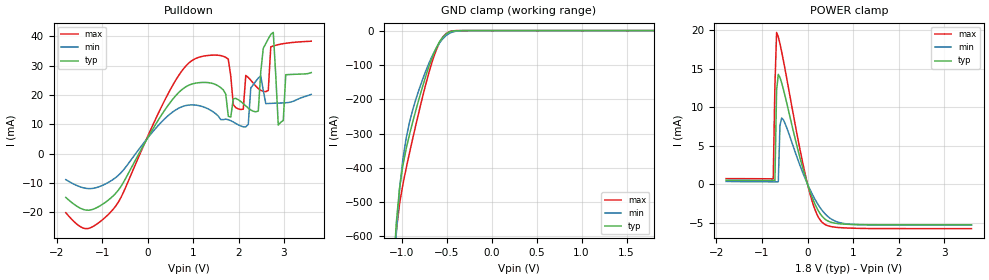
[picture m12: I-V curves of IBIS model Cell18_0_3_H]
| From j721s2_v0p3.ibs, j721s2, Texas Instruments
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|   Model Cell18_0_3_H
[Model]  Cell18_0_3_H
Model_type I/O_open_drain
Polarity   Non-Inverting
Enable   Active-High
Vinl =  0.540V
Vinh =  1.260V
Vmeas =  0.900V
Cref =  50.000pF
Rref =  1.000M
Vref =  0.0V
C_comp   8.808pF   8.664pF   8.912pF
[Model Spec]
Vinh   1.260V   1.134V   1.386V
Vinl   0.540V   0.486V   0.594V
Vmeas   0.900V   NA   NA
Vref   0.0V   NA   NA
Cref   50.000pF   NA   NA
Rref   1.000M   NA   NA
[Temperature Range]   25.000   0.125k   -40.000
[Voltage Range]   1.800V   1.620V   1.980V
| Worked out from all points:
|   slope of the pulldown table from 0 to 0.27 V, typ, clamps not added: 38.5 ohm
|   GND clamp passes 1 mA (typ) near -0.42 V on its own axis
|   POWER clamp passes 1 mA (typ) near -0.05 V on its own axis
[Pulldown]
|Voltage   I(typ)   I(min)   I(max)
-1.8V     -15mA      -8.914mA   -20.22mA
-755mV    -14.44mA   -8.818mA   -18.99mA
950mV     23.6mA     16.59mA    31.46mA
1.775V    12.73mA    11.55mA    32.22mA
2.05V     17.77mA    9.387mA    15.02mA
2.435V    14.5mA     25.77mA    22.19mA
2.545V    35.94mA    21.55mA    21.22mA
2.765V    41.37mA    17.16mA    36.74mA
2.875V    9.707mA    17.23mA    37.19mA
2.985V    11.28mA    17.29mA    37.52mA
3.04V     26.91mA    17.34mA    37.65mA
3.6V      27.63mA    20.2mA     38.36mA
[GND_clamp]
|Voltage   I(typ)   I(min)   I(max)
-1.8V     -12.3A     -11.29A    -13.31A
-1.097V   -731.7mA   -782.5mA   -731.7mA
-1.06V    -561.7mA   -593mA     -586mA
-1.023V   -458.8mA   -462.4mA   -504.6mA
-986mV    -392.6mA   -374mA     -448.2mA
-912mV    -302.1mA   -266.3mA   -355.6mA
-801mV    -193.6mA   -167.4mA   -229.4mA
-653mV    -73.19mA   -69.92mA   -84.18mA
-579mV    -32.5mA    -36.05mA   -34.84mA
-505mV    -9.453mA   -14.3mA    -8.331mA
-320mV    -33.8uA    -277.7uA   -6.183uA
1.8V      0A         0A         0A
[POWER_clamp]
|Voltage   I(typ)   I(min)   I(max)
-1.789V   502.3uA    344.3uA    709.8uA
-753mV    477.1uA    298.4uA    679.7uA
-716mV    477uA      297.5uA    12.77mA
-679mV    12.2mA     297.2uA    19.7mA
-642mV    14.25mA    301.9uA    19.14mA
-605mV    13.84mA    7.606mA    18.23mA
-568mV    13.14mA    8.59mA     17.18mA
-13mV     244.9uA    177.8uA    321.3uA
172mV     -2.72mA    -2.063mA   -3.44mA
320mV     -4.182mA   -3.407mA   -4.955mA
875mV     -5.218mA   -5.177mA   -5.702mA
3.6V      -5.284mA   -5.313mA   -5.786mA
[Ramp]
| variable   typ   min   max
dV/dt_r   0.541/0.227n   0.354/0.179n   0.705/0.288n
dV/dt_f   0.263/17.032n   0.114/15.169n   0.499/14.048n
R_load = 50.000
| ***************** End I2C 1.8V ****************************************
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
